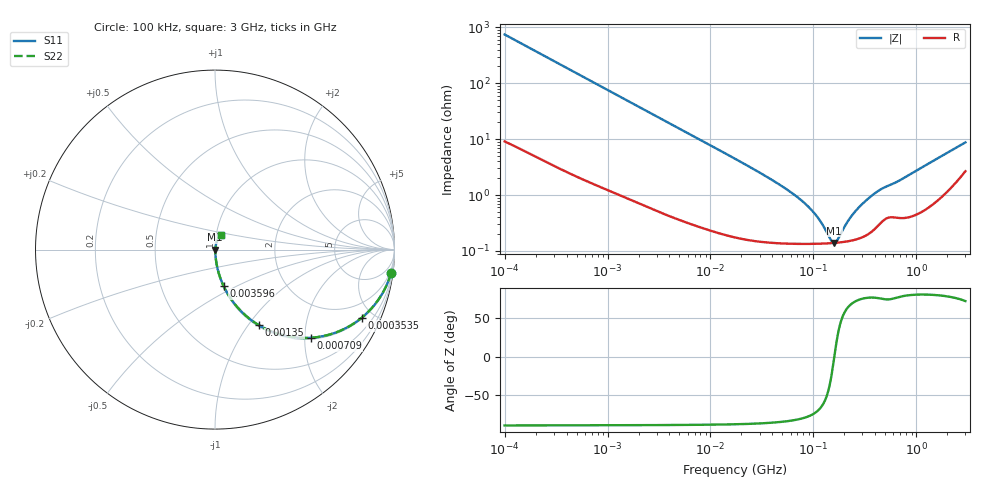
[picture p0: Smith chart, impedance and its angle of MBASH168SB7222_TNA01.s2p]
! MBASH168SB7222_TNA01  S-PARAMETER MODEL  ( Standard Model )
! Model Generated by TAIYO YUDEN Corporation (http://www.ty-top.com)
! Version 1.0
! TAIYO YUDEN Control No. 220601
! Copyright(c) 2013 TAIYO YUDEN CO.,LTD. All Rights Reserved.
! Product Description (link to TY-COMPAS)
! https://ds.yuden.co.jp/TYCOMPAS/or/detail?pn=MBASH168SB7222KTNA01&u=M
! Products Name : Multilayer Ceramic Capacitors
! Characteristics :
!  Capacitance : 2200 [pF] , Rated Voltage : 100 [V] , TCC : X7R
!  Case Size : 1.6 x 0.8 / 0.063 x 0.031 [mm/inch] , Thickness : 0.8 / 0.031 [mm/inch]
!  (Conditions: Temperature = 25 [degC] , DC Bias Voltage = 0 [V])
! External Node Assignments :
!  1  o---| |---o  2
! GND o---------o GND
! Frequency Range : 100kHz  -  3GHz  [ 401 STEP ]
# MHZ S RI R 50
! Freq[MHz].  S11 Real  S11 Imag  S21 Real  S21 Imag  S12 Real  S12 Imag  S22 Real  S22 Imag
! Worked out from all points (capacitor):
!   401 points, 100 kHz to 3 GHz, reference 50 ohm
!   read as one part in series: C = 2.13 nF near 105.3 kHz
!   lowest |Z| = 139 mohm at 158.9 MHz (marker M1)
!   series resonance near 159.8 MHz, so ESL is about 470 pH
!   S11 on the Smith chart (normalised r, x): 100 kHz: 1, -15; 353.5 kHz: 1.06, -4.26; 709 kHz: 1.03, -2.14; 1.35 MHz: 1.02, -1.13; 3.596 MHz: 1.01, -0.43; 3 GHz: 1.05, +0.17
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0.1  0.9808 -0.1313  0.0192 0.1313  0.0192 0.1313  0.9808 -0.1313
0.205778  0.9272 -0.2533  0.0728 0.2533  0.0728 0.2533  0.9272 -0.2533
0.353547  0.8164 -0.3805  0.1836 0.3805  0.1836 0.3805  0.8164 -0.3805
0.562235  0.6422 -0.4722  0.3578 0.4722  0.3578 0.4722  0.6422 -0.4722
0.709011  0.5329 -0.4914  0.4671 0.4914  0.4671 0.4914  0.5329 -0.4914
1.350433  0.2456 -0.4219  0.7544 0.4219  0.7544 0.4219  0.2456 -0.4219
2.039661  0.1282 -0.3251  0.8718 0.3251  0.8718 0.3251  0.1282 -0.3251
3.161081  0.0601 -0.2276  0.9399 0.2276  0.9399 0.2276  0.0601 -0.2276
3.595834  0.0478 -0.203  0.9522 0.203  0.9522 0.203  0.0478 -0.203
7.399428  0.0135 -0.103  0.9865 0.103  0.9865 0.103  0.0135 -0.103
17.7727  0.00361 -0.0433  0.9964 0.0433  0.9964 0.0433  0.00361 -0.0433
53.83243  0.00152 -0.0129  0.9985 0.0129  0.9985 0.0129  0.00152 -0.0129
97.38194  0.00136 -0.00507  0.9986 0.00507  0.9986 0.00507  0.00136 -0.00507
119.6798  0.00136 -0.00289  0.9986 0.00289  0.9986 0.00289  0.00136 -0.00289
147.0833  0.00138 -0.000819  0.9986 0.000819  0.9986 0.000819  0.00138 -0.000819
158.9065  0.00139 -5.49e-05  0.9986 5.49e-05  0.9986 5.49e-05  0.00139 -5.49e-05
171.6802  0.00141 0.00071  0.9986 -0.00071  0.9986 -0.00071  0.00141 0.00071
222.1509  0.00151 0.00333  0.9985 -0.00333  0.9985 -0.00333  0.00151 0.00333
280.1453  0.00171 0.00592  0.9983 -0.00592  0.9983 -0.00592  0.00171 0.00592
401.8672  0.00265 0.0106  0.9973 -0.0106  0.9973 -0.0106  0.00265 0.0106
547.5153  0.00418 0.0143  0.9958 -0.0143  0.9958 -0.0143  0.00418 0.0143
3000  0.0324 0.0786  0.9676 -0.0786  0.9676 -0.0786  0.0324 0.0786
